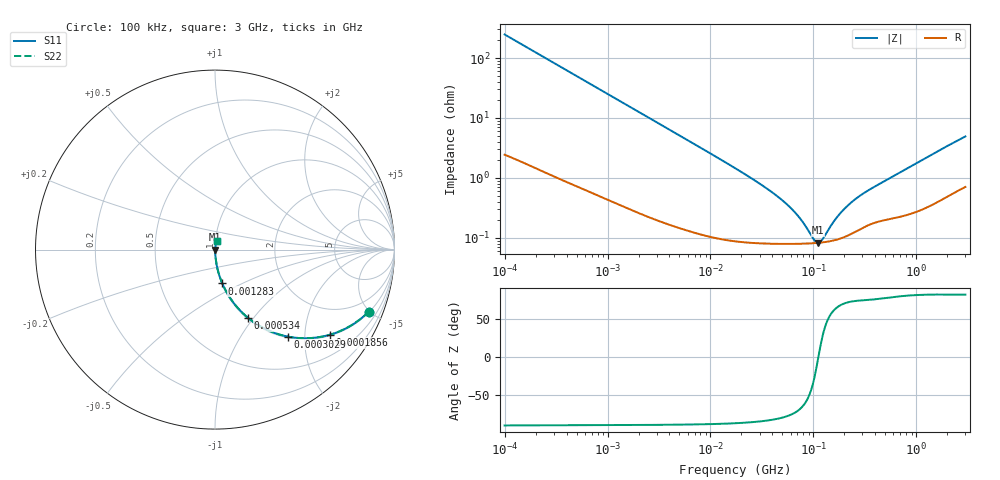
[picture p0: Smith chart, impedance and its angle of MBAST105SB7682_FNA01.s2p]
! MBAST105SB7682_FNA01  S-PARAMETER MODEL  ( Standard Model )
! Model Generated by TAIYO YUDEN Corporation (http://www.ty-top.com)
! Version 1.0
! TAIYO YUDEN Control No. 220601
! Copyright(c) 2013 TAIYO YUDEN CO.,LTD. All Rights Reserved.
! Product Description (link to TY-COMPAS)
! https://ds.yuden.co.jp/TYCOMPAS/or/detail?pn=MBAST105SB7682KFNA01&u=M
! Products Name : Multilayer Ceramic Capacitors
! Characteristics :
!  Capacitance : 6800 [pF] , Rated Voltage : 25 [V] , TCC : X7R
!  Case Size : 1.0 x 0.5 / 0.039 x 0.02 [mm/inch] , Thickness : 0.5 / 0.02 [mm/inch]
!  (Conditions: Temperature = 25 [degC] , DC Bias Voltage = 0 [V])
! External Node Assignments :
!  1  o---| |---o  2
! GND o---------o GND
! Frequency Range : 100kHz  -  3GHz  [ 401 STEP ]
# MHZ S RI R 50
! Freq[MHz].  S11 Real  S11 Imag  S21 Real  S21 Imag  S12 Real  S12 Imag  S22 Real  S22 Imag
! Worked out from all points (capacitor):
!   401 points, 100 kHz to 3 GHz, reference 50 ohm
!   read as one part in series: C = 6.42 nF near 105.3 kHz
!   lowest |Z| = 82.8 mohm at 110.8 MHz (marker M1)
!   series resonance near 111.8 MHz, so ESL is about 320 pH
!   S11 on the Smith chart (normalised r, x): 100 kHz: 1.05, -4.95; 185.6 kHz: 1.03, -2.68; 302.9 kHz: 1.02, -1.65; 534 kHz: 1.01, -0.94; 1.283 MHz: 1.01, -0.39; 3 GHz: 1.01, +0.10
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0.1  0.8571 -0.3451  0.1429 0.3451  0.1429 0.3451  0.8571 -0.3451
0.132776  0.7746 -0.4125  0.2254 0.4125  0.2254 0.4125  0.7746 -0.4125
0.185621  0.6403 -0.4742  0.3597 0.4742  0.3597 0.4742  0.6403 -0.4742
0.302894  0.4052 -0.4846  0.5948 0.4846  0.5948 0.4846  0.4052 -0.4846
0.533989  0.184 -0.3802  0.816 0.3802  0.816 0.3802  0.184 -0.3802
0.562235  0.1695 -0.3678  0.8305 0.3678  0.8305 0.3678  0.1695 -0.3678
0.82758  0.0883 -0.2757  0.9117 0.2757  0.9117 0.2757  0.0883 -0.2757
1.282589  0.0405 -0.1883  0.9595 0.1883  0.9595 0.1883  0.0405 -0.1883
3.161081  0.00832 -0.0798  0.9917 0.0798  0.9917 0.0798  0.00832 -0.0798
17.7727  0.00107 -0.0142  0.9989 0.0142  0.9989 0.0142  0.00107 -0.0142
34.73492  0.000848 -0.00673  0.9992 0.00673  0.9992 0.00673  0.000848 -0.00673
53.83243  0.000806 -0.0037  0.9992 0.0037  0.9992 0.0037  0.000806 -0.0037
73.34282  0.000801 -0.00202  0.9992 0.00202  0.9992 0.00202  0.000801 -0.00202
97.38194  0.000813 -0.000646  0.9992 0.000646  0.9992 0.000646  0.000813 -0.000646
105.21  0.00082 -0.000284  0.9992 0.000284  0.9992 0.000284  0.00082 -0.000284
110.7752  0.000826 -4.41e-05  0.9992 4.41e-05  0.9992 4.41e-05  0.000826 -4.41e-05
122.8043  0.000841 0.000437  0.9992 -0.000437  0.9992 -0.000437  0.000841 0.000437
167.3121  0.000933 0.00193  0.9991 -0.00193  0.9991 -0.00193  0.000933 0.00193
222.1509  0.00113 0.00344  0.9989 -0.00344  0.9989 -0.00344  0.00113 0.00344
310.5665  0.00153 0.00538  0.9985 -0.00538  0.9985 -0.00538  0.00153 0.00538
547.5153  0.00214 0.00956  0.9979 -0.00956  0.9979 -0.00956  0.00214 0.00956
3000  0.00935 0.0479  0.9906 -0.0479  0.9906 -0.0479  0.00935 0.0479
